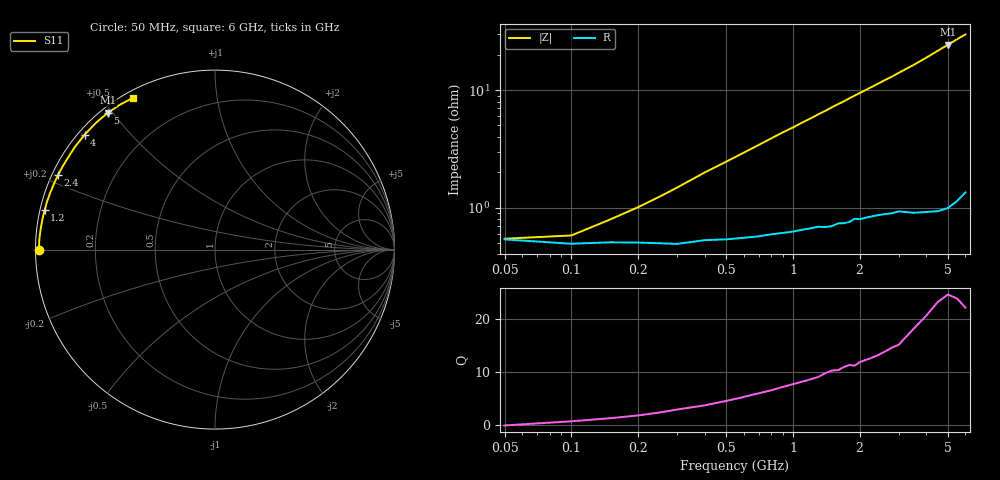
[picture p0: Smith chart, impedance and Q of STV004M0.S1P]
! SIEMENS Discrete & RF Semiconductors
! BA892
! Si PIN Diode in SCD-80
! IF = 4 mA
! S-Parameters:  September  1997
# GHz  S  MA  R  50
!  f  S11
! GHz  MAG  ANG
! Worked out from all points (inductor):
!   34 points, 50 MHz to 6 GHz, reference 50 ohm
!   read as one part to ground: L = 765 pH near 400 MHz
!   highest Q = 23.8 at 5 GHz (marker M1), where L = 774 pH
!   S11 on the Smith chart (normalised r, x): 50 MHz: 0.01, -0.00; 1.2 GHz: 0.01, +0.11; 2.4 GHz: 0.02, +0.22; 4 GHz: 0.02, +0.38; 5 GHz: 0.02, +0.49; 6 GHz: 0.03, +0.59
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0.05  0.9788 -179.8
0.1  0.9805 179.3
0.15  0.9799 178.6
0.3  0.9806 176.8
0.4  0.9791 175.6
0.6  0.9782 173.4
0.8  0.9767 171.2
0.9  0.9761 170.1
1.2  0.974 167.0
1.3  0.9733 165.9
1.4  0.9735 164.9
1.5  0.973 163.8
1.6  0.9717 162.8
1.7  0.9717 161.8
1.8  0.9711 160.7
1.9  0.9693 159.7
2  0.9697 158.7
2.2  0.9686 156.7
2.4  0.9678 154.7
2.6  0.9673 152.7
2.8  0.967 150.8
3  0.9661 148.7
3.5  0.9678 143.8
4  0.9684 138.6
4.5  0.969 133.3
5  0.9685 128.1
5.5  0.9654 123.1
6  0.961 118.5
